(* Simple derived node - always returns FAILURE *)
FUNCTION_BLOCK FB_AlwaysFailure EXTENDS FB_BaseNode

METHOD Tick : E_NodeStatus
Tick := E_NodeStatus.FAILURE;
eLastStatus := E_NodeStatus.FAILURE;
END_METHOD

END_FUNCTION_BLOCK
